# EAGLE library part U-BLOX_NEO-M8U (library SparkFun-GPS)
u-blox NEO-M8U The NEO-M8U module introduces u-blox’s Untethered Dead Reckoning (UDR) technology, which provides continuous navigation without requiring speed information from the vehicle. This innovative technology brings the benefits of dead reckoning to installations previously restricted to using GNSS alone, and significantly reduces the cost of installation for after-market dead reckoning applications. The strength of UDR is particularly apparent under poor signal conditions, where it brings continuous positioning in urban environments, even to devices with antennas installed within the vehicle. Useful positioning performance is also available during complete signal loss, for example in parking garages and short tunnels. With UDR, positioning starts as soon as power is applied to the module, before the first GNSS fix is available. The NEO-M8U may be installed in any position within the vehicle without configuration. In addition to its freedom from any electrical connection to the vehicle, the on-board accelerometer and gyroscope sensors result in a fully self-contained solution, perfect for rapid product development with reliable and consistent performance.
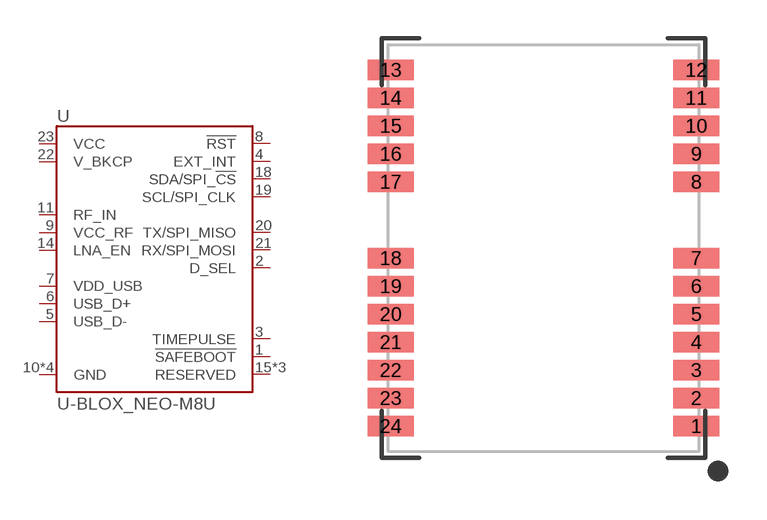
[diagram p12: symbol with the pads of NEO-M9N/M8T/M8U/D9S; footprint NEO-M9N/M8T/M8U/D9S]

Designator prefix U

## U-BLOX_NEO-M8U (PROD_ID: IC-14850)  [NEO-M9N/M8T/M8U/D9S]
1  !SAFEBOOT!
2  D_SEL
3  TIMEPULSE
4  EXT_INT
5  USB_D-
6  USB_D+
7  VDD_USB
8  !RST
9  VCC_RF
10  GND
11  RF_IN
12  GND
13  GND
14  LNA_EN
15  RESERVED  nc
16  RESERVED  nc
17  RESERVED  nc
18  SDA/SPI_!CS!
19  SCL/SPI_CLK
20  TX/SPI_MISO
21  RX/SPI_MOSI
22  V_BKCP
23  VCC
24  GND

## Footprint NEO-M9N/M8T/M8U/D9S (pad centres in mm)
u-blox NEO-M9N/M8T/M8U/D9S Module Mechanical Specifications Overall: 12.2mm x 16.0mm Pad Pitch: 1.1mm Pad Width: .8mm Pad Length: .9mm Number of Pins: 24
smd 1.8 x 0.8: 1 6,-7; 2 6,-5.9; 3 6,-4.8; 4 6,-3.7; 5 6,-2.6; 6 6,-1.5; 7 6,-0.4; 8 6,2.6; 9 6,3.7; 10 6,4.8; 11 6,5.9; 12 6,7; 13 -6,7; 14 -6,5.9; 15 -6,4.8; 16 -6,3.7; 17 -6,2.6; 18 -6,-0.4; 19 -6,-1.5; 20 -6,-2.6; 21 -6,-3.7; 22 -6,-4.8; 23 -6,-5.9; 24 -6,-7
